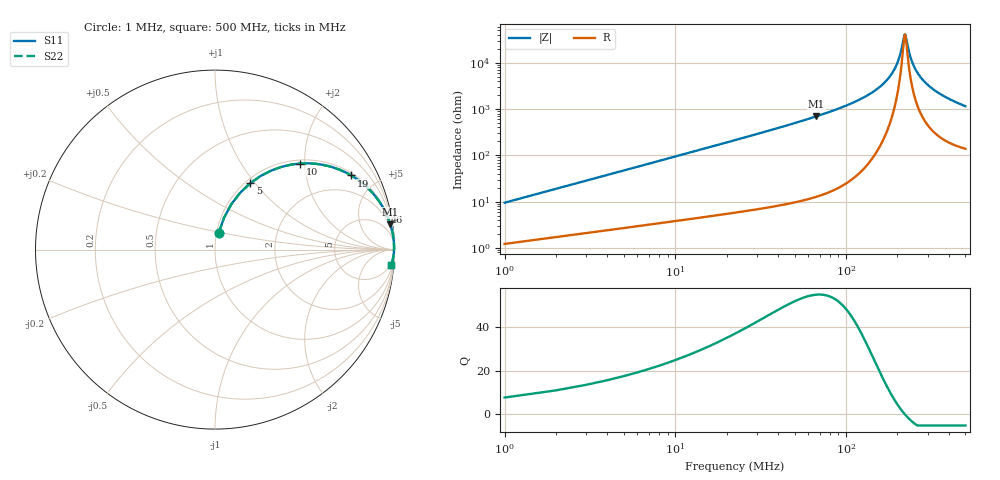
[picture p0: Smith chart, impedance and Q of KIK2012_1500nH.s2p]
!version-2
!date-01.2022
!Series
# MHz S RI R 50
!Freq ReS11 ImS11 ReS21 ImS21 ReS12 ImS12 ReS22 ImS22
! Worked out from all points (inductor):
!   500 points, 1 MHz to 500 MHz, reference 50 ohm
!   read as one part in series: L = 1.5 uH near 3 MHz
!   highest Q = 54.5 at 67 MHz (marker M1), where L = 1.65 uH
!   self-resonance near 221 MHz
!   S11 on the Smith chart (normalised r, x): 1 MHz: 1.02, +0.19; 5 MHz: 1.05, +0.94; 10 MHz: 1.08, +1.89; 19 MHz: 1.11, +3.61; 46 MHz: 1.18, +9.06; 500 MHz: 4, -23
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1  0.0206 0.0912  0.9794 -0.0912  0.9794 -0.0912  0.0206 0.0912
5  0.1958 0.3692  0.8042 -0.3692  0.8042 -0.3692  0.1958 0.3692
10  0.4729 0.4795  0.5271 -0.4795  0.5271 -0.4795  0.4729 0.4795
14  0.6329 0.4652  0.3671 -0.4652  0.3671 -0.4652  0.6329 0.4652
19  0.7587 0.4134  0.2413 -0.4134  0.2413 -0.4134  0.7587 0.4134
29  0.8797 0.3135  0.1203 -0.3135  0.1203 -0.3135  0.8797 0.3135
46  0.9498 0.2086  0.0502 -0.2086  0.0502 -0.2086  0.9498 0.2086
67  0.9773 0.1402  0.0227 -0.1402  0.0227 -0.1402  0.9773 0.1402
85  0.9869 0.1048  0.0131 -0.1048  0.0131 -0.1048  0.9869 0.1048
168  0.9975 0.0267  0.0025 -0.0267  0.0025 -0.0267  0.9975 0.0267
186  0.9978 0.0167  0.00225 -0.0167  0.00225 -0.0167  0.9978 0.0167
199  0.9978 0.0102  0.00223 -0.0102  0.00223 -0.0102  0.9978 0.0102
207  0.9977 0.00642  0.00228 -0.00642  0.00228 -0.00642  0.9977 0.00642
218  0.9976 0.00149  0.0024 -0.00149  0.0024 -0.00149  0.9976 0.00149
221  0.9976 0.000187  0.00244 -0.000187  0.00244 -0.000187  0.9976 0.000187
224  0.9975 -0.0011  0.00249 0.0011  0.00249 0.0011  0.9975 -0.0011
237  0.9973 -0.00647  0.00275 0.00647  0.00275 0.00647  0.9973 -0.00647
251  0.9969 -0.0119  0.0031 0.0119  0.0031 0.0119  0.9969 -0.0119
284  0.9958 -0.0238  0.0042 0.0238  0.0042 0.0238  0.9958 -0.0238
334  0.9936 -0.0399  0.00644 0.0399  0.00644 0.0399  0.9936 -0.0399
417  0.9886 -0.0632  0.0114 0.0632  0.0114 0.0632  0.9886 -0.0632
500  0.9825 -0.0838  0.0175 0.0838  0.0175 0.0838  0.9825 -0.0838
